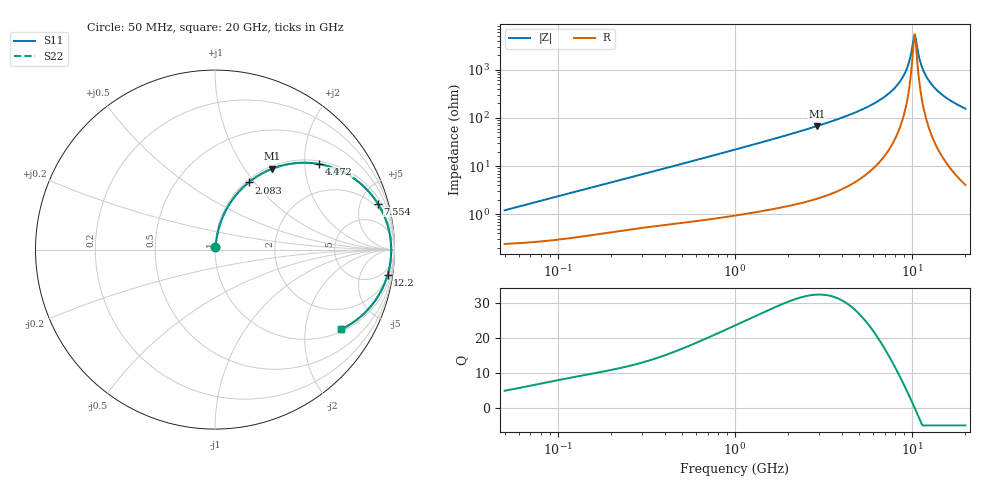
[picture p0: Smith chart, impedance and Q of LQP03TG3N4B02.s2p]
!Murata Part Number: LQP03TG3N4B02
!These Parameters are Measured in Series Mode Connection
!  o--[Z]--o
!Port1  Port2
!  o-------o
!Freq. Start=50[MHz] Stop=20[GHz], 401[Steps]
# Hz S RI R 50
!Freq.(Hz) S11(Real) S11(Imag) S21(Real) S21(Imag) S12(Real) S12(Imag) S22(Real) S22(Imag)
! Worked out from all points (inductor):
!   401 points, 50 MHz to 20 GHz, reference 50 ohm
!   read as one part in series: L = 3.75 nH near 51.52 MHz
!   highest Q = 32.3 at 2.896 GHz (marker M1), where L = 3.71 nH
!   self-resonance near 10.35 GHz
!   S11 on the Smith chart (normalised r, x): 50 MHz: 1.00, +0.02; 2.083 GHz: 1.03, +0.94; 4.472 GHz: 1.08, +2.35; 7.554 GHz: 1.49, +6.89; 12.2 GHz: 3, -13; 20 GHz: 1.08, -3.13
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5e7  0.00255 0.0118  0.9975 -0.0118  0.9975 -0.0118  0.00255 0.0118
1.364002e8  0.00441 0.0314  0.9956 -0.0314  0.9956 -0.0314  0.00441 0.0314
3.721004e8  0.0125 0.0816  0.9875 -0.0816  0.9875 -0.0816  0.0125 0.0816
1e9  0.0541 0.206  0.9459 -0.206  0.9459 -0.206  0.0541 0.206
2.083303e9  0.1874 0.3743  0.8126 -0.3743  0.8126 -0.3743  0.1874 0.3743
2.728004e9  0.29 0.4385  0.71 -0.4385  0.71 -0.4385  0.29 0.4385
2.896447e9  0.3182 0.4506  0.6818 -0.4506  0.6818 -0.4506  0.3182 0.4506
4.472136e9  0.5786 0.4769  0.4214 -0.4769  0.4214 -0.4769  0.5786 0.4769
5.944466e9  0.7727 0.3973  0.2273 -0.3973  0.2273 -0.3973  0.7727 0.3973
7.442007e9  0.9003 0.2672  0.0997 -0.2672  0.0997 -0.2672  0.9003 0.2672
7.554318e9  0.9071 0.2567  0.0929 -0.2567  0.0929 -0.2567  0.9071 0.2567
8.389408e9  0.9474 0.1773  0.0526 -0.1773  0.0526 -0.1773  0.9474 0.1773
9.041845e9  0.9672 0.1159  0.0328 -0.1159  0.0328 -0.1159  0.9672 0.1159
9.457416e9  0.9752 0.0778  0.0248 -0.0778  0.0248 -0.0778  0.9752 0.0778
1.004137e10  0.981 0.0261  0.019 -0.0261  0.019 -0.0261  0.981 0.0261
1.034674e10  0.9819 3.83e-05  0.0181 -3.83e-05  0.0181 -3.83e-05  0.9819 3.83e-05
1.066139e10  0.9813 -0.026  0.0187 0.026  0.0187 0.026  0.9813 -0.026
1.131968e10  0.9761 -0.0779  0.0239 0.0779  0.0239 0.0779  0.9761 -0.0779
1.220001e10  0.9618 -0.1413  0.0382 0.1413  0.0382 0.1413  0.9618 -0.1413
1.334722e10  0.9341 -0.2135  0.0659 0.2135  0.0659 0.2135  0.9341 -0.2135
1.482269e10  0.8886 -0.2899  0.1114 0.2899  0.1114 0.2899  0.8886 -0.2899
2e10  0.7048 -0.4434  0.2952 0.4434  0.2952 0.4434  0.7048 -0.4434
